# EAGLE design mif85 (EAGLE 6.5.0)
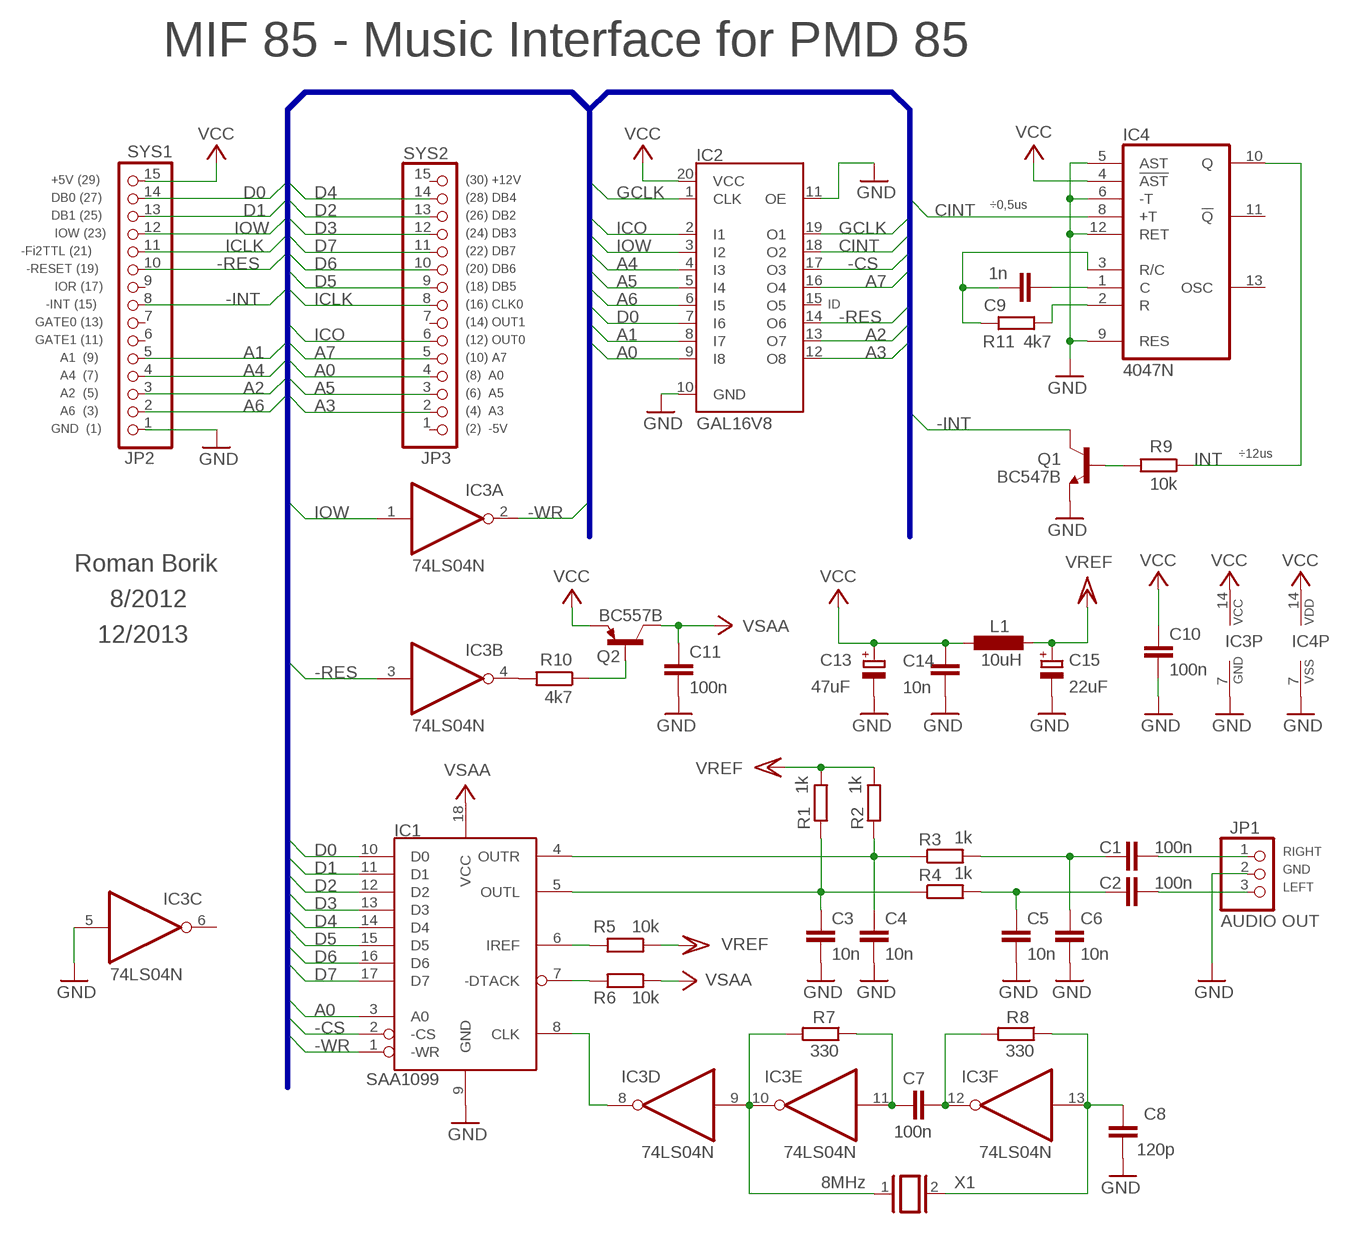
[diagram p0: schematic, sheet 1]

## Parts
C1  100n  C-EU025-025X050  [C025-025X050]
C2  100n  C-EU025-025X050  [C025-025X050]
C3  10n  C-EU025-025X050  [C025-025X050]
C4  10n  C-EU025-025X050  [C025-025X050]
C5  10n  C-EU025-025X050  [C025-025X050]
C6  10n  C-EU025-025X050  [C025-025X050]
C7  100n  C-EU025-025X050  [C025-025X050]
C8  120p  C-EU025-025X050  [C025-025X050]
C9  1n  C-EU025-025X050  [C025-025X050]
C10  100n  C-EU025-025X050  [C025-025X050]
C11  100n  C-EU025-025X050  [C025-025X050]
C13  47uF  CPOL-EUE2,5-6E  [E2,5-6E]
C14  10n  C-EU025-025X050  [C025-025X050]
C15  22uF  CPOL-EUE2,5-6E  [E2,5-6E]
IC1  SAA1099  [DIL18]
IC2  GAL16V8  ATF16V8BP3  [DIL20]
IC3  74LS04N  [DIL14]
IC4  4047N  [DIL14]
JP1  AUDIO OUT  PINHD-1X3  [1X03]
JP2  SYS1  PINHD-1X15  [1X15]
JP3  SYS2  PINHD-1X15  [1X15]
L1  10uH  L-EU0207/7  [0207/7]
Q1  BC547B  [TO92]
Q2  BC557B  BC557  [TO92]
R1  1k  R-EU_0207/7  [0207/7]
R2  1k  R-EU_0207/7  [0207/7]
R3  1k  R-EU_0207/7  [0207/7]
R4  1k  R-EU_0207/7  [0207/7]
R5  10k  R-EU_0207/7  [0207/7]
R6  10k  R-EU_0207/7  [0207/7]
R7  330  R-EU_0207/7  [0207/7]
R8  330  R-EU_0207/7  [0207/7]
R9  10k  R-EU_0207/7  [0207/7]
R10  4k7  R-EU_0207/7  [0207/7]
R11  4k7  R-EU_0207/7  [0207/7]
X1  8MHz  XTAL/S  [QS]

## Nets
-CS: IC1.2(-CS) IC2.17(O3)
-INT: JP2.8 Q1.3(C)
-RES: IC2.14(O6) IC3.3(B:I) JP2.10
-WR: IC1.1(-WR) IC3.2(A:O)
A0: IC1.3(A0) IC2.9(I8) JP3.4
A1: IC2.8(I7) JP2.5
A2: IC2.13(O7) JP2.3
A3: IC2.12(O8) JP3.2
A4: IC2.4(I3) JP2.4
A5: IC2.5(I4) JP3.3
A6: IC2.6(I5) JP2.2
A7: IC2.16(O4) JP3.5
CINT: IC2.18(O2) IC4.8(+T)
D0: IC1.10(D0) IC2.7(I6) JP2.14
D1: IC1.11(D1) JP2.13
D2: IC1.12(D2) JP3.13
D3: IC1.13(D3) JP3.12
D4: IC1.14(D4) JP3.14
D5: IC1.15(D5) JP3.9
D6: IC1.16(D6) JP3.10
D7: IC1.17(D7) JP3.11
GCLK: IC2.1(CLK) IC2.19(O1)
GND: C3.2 C4.2 C5.2 C6.2 C8.2 C10.2 C11.2 C13.- C14.2 C15.- IC1.9(GND) IC2.10(GND) IC2.11(OE) IC3.5(C:I) IC3.7(P:GND) IC4.5(AST) IC4.6(-T) IC4.7(VSS) IC4.9(RES) IC4.12(RET) JP1.2 JP2.1 Q1.1(E)
ICLK: JP2.11 JP3.8
ICO: IC2.2(I1) JP3.6
INT: IC4.10(Q) R9.2
IOW: IC2.3(I2) IC3.1(A:I) JP2.12
N$1: IC3.9(D:I) IC3.10(E:O) R7.2 X1.1
N$2: C7.1 IC3.12(F:O) R8.2
N$3: C7.2 IC3.11(E:I) R7.1
N$4: Q1.2(B) R9.1
N$5: C8.1 IC3.13(F:I) R8.1 X1.2
N$6: IC1.8(CLK) IC3.8(D:O)
N$7: IC4.2(R) R11.2
N$8: IC3.4(B:O) R10.2
N$9: Q2.2(B) R10.1
N$10: IC1.7(-DTACK) R6.2
N$11: IC1.6(IREF) R5.2
N$12: C4.1 IC1.4(OUTR) R2.1 R3.1
N$13: C3.1 IC1.5(OUTL) R1.1 R4.1
N$14: C2.1 C5.1 R4.2
N$15: C1.1 C6.1 R3.2
N$16: C2.2 JP1.3
N$17: C1.2 JP1.1
N$18: C9.2 IC4.1(C)
N$19: C9.1 IC4.3(R/C) R11.1
V+: C11.1 IC1.18(VCC) Q2.3(C) R6.1 ; supply symbol labelled VSAA
VCC: C10.1 C13.+ C14.1 IC2.20(VCC) IC3.14(P:VCC) IC4.4(!AST) IC4.14(VDD) JP2.15 L1.2 Q2.1(E)
VREF: C15.+ L1.1 R1.2 R2.2 R5.1
Unconnected: IC2.15(O5) IC3.6(C:O) IC4.11(!Q) IC4.13(OSC) JP2.6 JP2.7 JP2.9 JP3.1 JP3.7 JP3.15

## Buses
SYS:D[0..7],A[0..7],IOW,-INT,-RES,ICO,ICLK,GCLK,-CS,-WR,CINT

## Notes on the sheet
- MIF 85 - Music Interface for PMD 85
- +5V (29) | (30) +12V
- DB0 (27) | (28) DB4
- ÷0,5us
- DB1 (25) | (26) DB2
- IOW (23) | (24) DB3
- -Fi2TTL (21) | (22) DB7
- -RESET (19) | (20) DB6
- IOR (17) | (18) DB5
- -INT (15) | (16) CLK0 | ID
- GATE0 (13) | (14) OUT1
- GATE1 (11) | (12) OUT0
- A1  (9) | (10) A7
- A4  (7) | (8)  A0
- A2  (5) | (6)  A5
- A6  (3) | (4)  A3
- GND  (1) | (2)  -5V
- ÷12us
- Roman Borik
- 8/2012
- 12/2013
- RIGHT
- GND
- LEFT

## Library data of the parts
C1-C11 C14 = rcl:C-EU: CAPACITOR, European symbol
C13 C15 = rcl:CPOL-EU: POLARIZED CAPACITOR, European symbol
IC1 = rombor:SAA1099
IC2 = atmel:ATF16V8B: High perfomance CMOS (electrically erasable) programmable logic device (PLD) ABLE-Atmel-ABEL - P18V8R, P16V8C, P16V8AS, P17V8 COPL Atmel-WinCUPL - G16V8MS, G16V8MA, G16V8AS, G16V8 LOG/IC - GAL16V8_R, GAL16V8_G7, GAL16V8_C), GAL16V8 Tango-PLD - G16V8R, G16V8C, G16V8AS, G16V8 Source: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; MPN: ATF16V8CZ-15PU; OC_FARNELL: 1551768; OC_NEWARK: 94M6254
IC3 = 74xx-eu:74*04: Hex INVERTER
IC4 = 40xx:4047: LP monostable/astable MULTIVIBRATOR
JP1 = pinhead:PINHD-1X3: PIN HEADER
JP2 JP3 = pinhead:PINHD-1X15: PIN HEADER
L1 = rcl:L-EU: INDUCTOR, European symbol
Q1 = transistor-npn:BC547*: NPN Transistor
Q2 = transistor-pnp:BC557: PNP Transistor
R1-R11 = rcl:R-EU_: RESISTOR, European symbol
X1 = special:XTAL/S: CRYSTAL

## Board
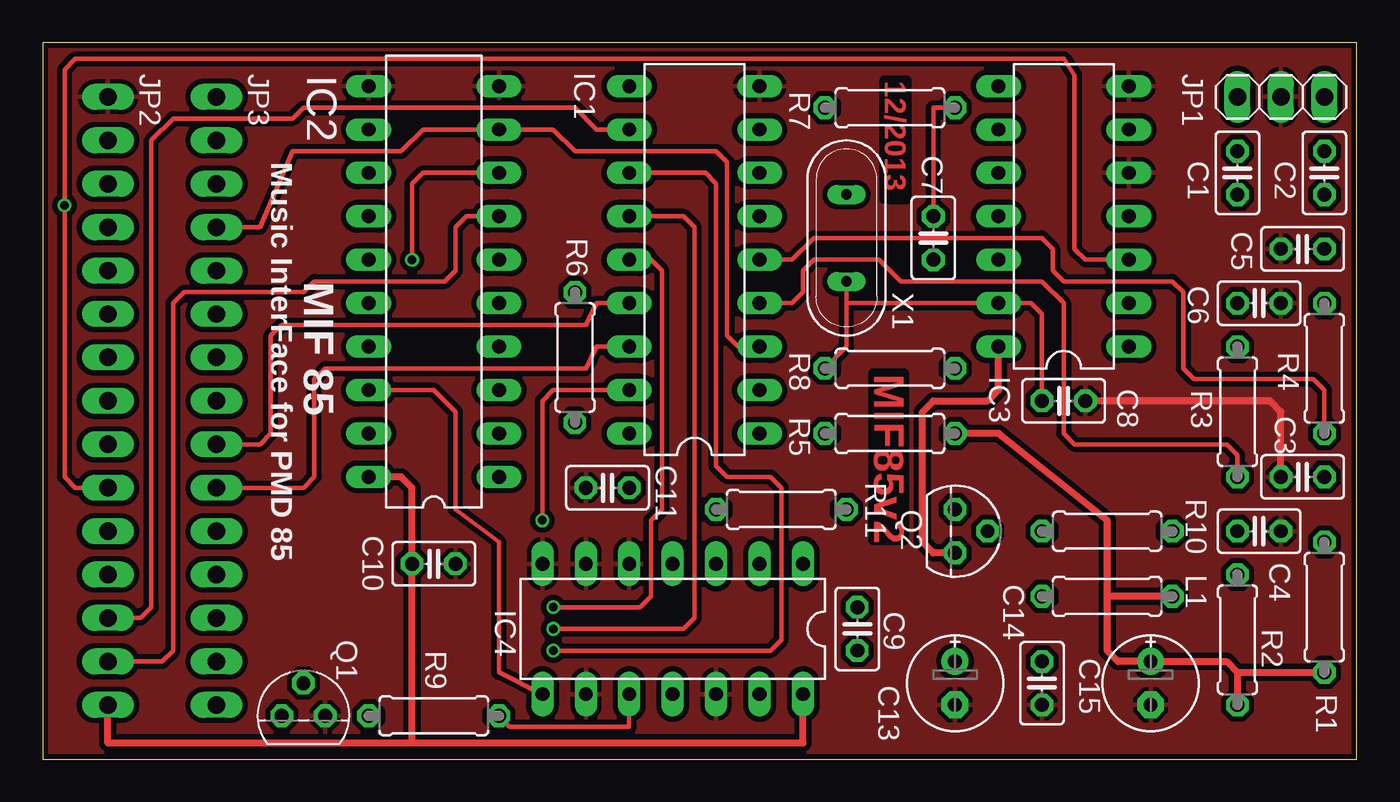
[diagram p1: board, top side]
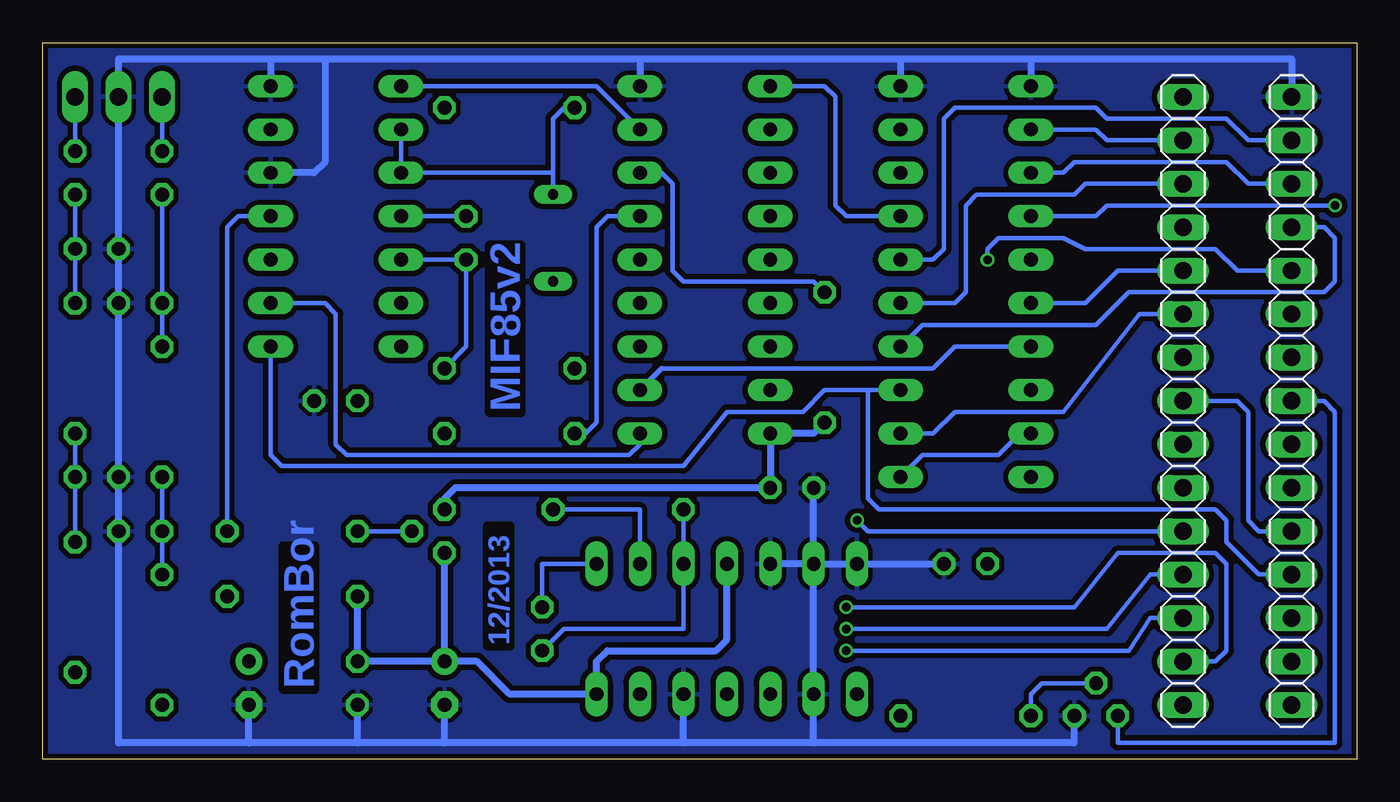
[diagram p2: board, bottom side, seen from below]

Size 76.82 x 41.9 mm. Coordinates in mm from the lower left corner, seen from the top.
Outline: 0,0 76.82,0 76.82,41.9 0,41.9 0,0
Copper layers (1*16): Top 0.035mm / dielectric 1.5mm / Bottom 0.035mm
Design rules "SeeedStudio_2layer_DRU_no_angle_20140221": minimum track width 6mil, minimum drill 12mil, track to track 6mil, track to pad 6mil, pad to pad 6mil, via to via 6mil, smd to smd 0mil, copper to edge 10mil, drill to drill 10mil, minimum pad ring 10mil, minimum via ring 6mil, stop-mask expansion 2mil, vias tented up to drill 100mil, thermal gap 10mil

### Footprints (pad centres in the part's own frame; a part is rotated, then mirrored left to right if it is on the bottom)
C025-025X050 = drill 0.813 octagon: 1 -1.27,0; 2 1.27,0
E2,5-6E = drill 0.813 pad 1.575: + -1.27,0 | drill 0.813 pad 1.575 octagon: - 1.27,0
DIL18 = drill 0.813 long: 1 -10.16,-3.81; 2 -7.62,-3.81; 3 -5.08,-3.81; 4 -2.54,-3.81; 5 0,-3.81; 6 2.54,-3.81; 7 5.08,-3.81; 8 7.62,-3.81; 9 10.16,-3.81; 10 10.16,3.81; 11 7.62,3.81; 12 5.08,3.81; 13 2.54,3.81; 14 0,3.81; 15 -2.54,3.81; 16 -5.08,3.81; 17 -7.62,3.81; 18 -10.16,3.81
DIL20 = drill 0.813 long: 1 -11.43,-3.81; 2 -8.89,-3.81; 3 -6.35,-3.81; 4 -3.81,-3.81; 5 -1.27,-3.81; 6 1.27,-3.81; 7 3.81,-3.81; 8 6.35,-3.81; 9 8.89,-3.81; 10 11.43,-3.81; 11 11.43,3.81; 12 8.89,3.81; 13 6.35,3.81; 14 3.81,3.81; 15 1.27,3.81; 16 -1.27,3.81; 17 -3.81,3.81; 18 -6.35,3.81; 19 -8.89,3.81; 20 -11.43,3.81
DIL14 = drill 0.813 long: 1 -7.62,-3.81; 2 -5.08,-3.81; 3 -2.54,-3.81; 4 0,-3.81; 5 2.54,-3.81; 6 5.08,-3.81; 7 7.62,-3.81; 8 7.62,3.81; 9 5.08,3.81; 10 2.54,3.81; 11 0,3.81; 12 -2.54,3.81; 13 -5.08,3.81; 14 -7.62,3.81
1X03 = drill 1.016 long: 1 -2.54,0; 2 0,0; 3 2.54,0
1X15 = drill 1.016 long: 1 -17.78,0; 2 -15.24,0; 3 -12.7,0; 4 -10.16,0; 5 -7.62,0; 6 -5.08,0; 7 -2.54,0; 8 0,0; 9 2.54,0; 10 5.08,0; 11 7.62,0; 12 10.16,0; 13 12.7,0; 14 15.24,0; 15 17.78,0
0207/7 = drill 0.813 octagon: 1 -3.81,0; 2 3.81,0
TO92 = drill 0.813 octagon: 1 1.27,0; 2 0,1.905; 3 -1.27,0
QS = drill 0.61 long: 1 -2.54,0; 2 2.54,0

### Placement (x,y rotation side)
C1  69.85,34.29 90 top
C2  74.93,34.29 90 top
C3  73.66,16.51 180 top
C4  71.12,13.34 0 top
C5  73.66,29.84 180 top
C6  71.12,26.67 0 top
C7  52.07,30.48 90 top
C8  59.69,20.95 0 top
C9  47.62,7.62 90 top
C10  22.86,11.43 0 top
C11  33.02,15.88 180 top
C13  53.34,4.45 270 top
C14  58.42,4.45 270 top
C15  64.77,4.45 270 top
IC1  38.1,29.21 90 top
IC2  22.86,27.94 90 top
IC3  59.69,31.75 90 top
IC4  36.83,7.62 180 top
JP1  72.39,38.73 0 top
JP2  3.81,20.95 270 bottom
JP3  10.16,20.95 270 bottom
L1  62.23,9.53 180 top
Q1  15.24,2.54 0 top
Q2  53.34,13.34 270 top
R1  74.93,8.89 270 top
R2  69.85,6.99 270 top
R3  69.85,20.32 90 top
R4  74.93,22.86 90 top
R5  49.53,19.05 180 top
R6  31.11,23.5 90 top
R7  49.53,38.1 180 top
R8  49.53,22.86 0 top
R9  22.86,2.54 0 top
R10  62.23,13.34 0 top
R11  43.18,14.61 0 top
X1  46.99,30.48 270 top

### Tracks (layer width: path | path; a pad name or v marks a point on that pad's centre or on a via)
-CS
  Bottom 0.254: IC2.17 23.5,24.13 24.77,22.86 40.64,22.86
  Bottom 0.305: 40.64,22.86 IC1.2
-INT
  Bottom 0.254: JP2.8 1.91,20.95 1.27,20.32 1.27,0.95 13.97,0.95 Q1.3
-RES  (via drill 0.5)
  Top 0.254: IC3.3 60.96,29.21 60.33,29.84 60.33,40.01 59.69,40.96 1.91,40.96 1.27,40.32 v1.27,32.38 1.27,16.51 1.91,15.88 JP2.10
  Bottom 0.254: IC2.14 15.24,31.75 14.61,32.38 v1.27,32.38
-WR
  Bottom 0.254: IC1.1 41.91,18.41 42.55,17.78 59.05,17.78 59.69,18.41 59.69,26.04 60.33,26.67 IC3.2
A0
  Top 0.254: JP3.4 12.7,31.11 14.61,35.56 20.95,35.56 22.23,36.83 IC2.9 29.84,36.83 31.11,35.56 39.37,35.56 40.01,34.92 40.01,24.77 40.64,24.13 IC1.3
A1  (via drill 0.5)
  Top 0.254: v21.59,29.21 21.59,33.66 22.23,34.29 IC2.8
  Bottom 0.254: v21.59,29.21 21.59,29.84 20.95,30.48 17.14,30.48 15.88,29.84 8.26,29.84 6.99,28.57 JP2.5
A2
  Bottom 0.254: JP2.3 6.35,33.66 7.62,34.92 16.51,34.92 17.14,34.29 IC2.13
A3
  Bottom 0.254: JP3.2 14.61,36.2 15.24,36.83 IC2.12
A4
  Bottom 0.254: JP2.4 1.91,31.11 1.27,30.48 1.27,27.94 1.91,27.3 13.34,27.3 15.24,25.4 25.4,25.4 IC2.4
A5
  Bottom 0.254: IC2.5 23.5,26.67 22.86,27.3 22.86,32.38 22.23,33.02 16.51,33.02 15.88,33.66 JP3.3
A6
  Bottom 0.254: JP2.2 6.35,36.2 7.62,37.47 14.61,37.47 15.24,38.1 23.5,38.1 24.13,37.47 24.13,29.84 24.77,29.21 IC2.6
A7
  Bottom 0.254: JP3.5 13.97,28.57 15.88,26.67 IC2.16
CINT
  Top 0.254: IC4.8 26.67,5.08 26.67,12.7 24.13,14.61 24.13,20.32 22.86,21.59 IC2.18
D0
  Top 0.254: IC2.7 24.77,31.75 24.13,31.11 24.13,28.57 23.5,27.94 15.88,27.94 15.24,27.3 8.26,27.3 7.62,26.67 7.62,6.35 6.99,5.71 JP2.14
  Bottom 0.254: IC1.10 31.11,39.37 30.48,38.73 30.48,32.38 29.84,31.75 IC2.7
D1
  Top 0.254: IC1.11 32.38,36.83 31.11,38.1 15.24,38.1 14.61,37.47 7.62,37.47 6.35,36.2 6.35,8.89 5.71,8.26 JP2.13
D2  (via drill 0.5)
  Top 0.254: IC1.12 38.73,34.29 39.37,33.66 39.37,17.14 40.01,16.51 42.55,16.51 43.18,15.88 43.18,6.99 42.55,6.35 v29.84,6.35
  Bottom 0.254: v29.84,6.35 13.34,6.35 12.06,8.26 JP3.13
D3  (via drill 0.5)
  Top 0.254: IC1.13 37.47,31.75 38.1,31.11 38.1,8.26 37.47,7.62 v29.84,7.62
  Bottom 0.254: v29.84,7.62 14.61,7.62 12.06,10.79 JP3.12
D4  (via drill 0.5)
  Top 0.254: 35.56,29.21 36.2,28.57 36.2,14.61 35.56,13.97 35.56,9.53 34.92,8.89 v29.84,8.89
  Top 0.305: 35.56,29.21 IC1.14
  Bottom 0.254: v29.84,8.89 16.51,8.89 13.97,12.06 8.26,12.06 7.62,11.43 7.62,6.35 8.26,5.71 JP3.14
D5
  Top 0.254: IC1.15 32.38,26.67 31.75,25.4 13.97,25.4 13.34,24.77 13.34,19.05 12.7,18.41 JP3.9
D6
  Top 0.254: IC1.16 32.38,24.13 31.75,22.86 16.51,22.86 15.88,22.23 15.88,16.51 15.24,15.88 JP3.10
D7  (via drill 0.5)
  Top 0.254: IC1.17 29.84,21.59 29.21,20.95 v29.21,13.97
  Bottom 0.254: v29.21,13.97 28.57,13.34 JP3.11
GCLK
  Bottom 0.254: IC2.1 25.4,17.78 20.95,17.78 19.68,19.05 IC2.19
GND
  Top 0.406: C8.2 71.75,20.95 72.39,20.32 C3.2
  Bottom 0.406: 64.77,0.95 72.39,0.95 C4.2 C3.2 C6.2 C5.2 JP1.2 72.39,40.96 63.5,40.96 | 63.5,40.96 IC3.7 | 63.5,40.96 60.33,40.96 | 60.33,40.96 60.33,34.92 60.96,34.29 IC3.5 | 60.33,40.96 41.91,40.96 | 41.91,40.96 IC1.9 | 41.91,40.96 26.67,40.96 | 26.67,40.96 IC2.10 | 26.67,40.96 19.05,40.96 | 19.05,40.96 IC2.11 | 19.05,40.96 3.81,40.96 JP2.1 | 64.77,0.95 C15.- | 58.42,0.95 64.77,0.95 | 58.42,0.95 C14.2 | 53.34,0.95 58.42,0.95 | 53.34,0.95 C13.- | 39.37,0.95 53.34,0.95 | 39.37,0.95 IC4.12 | 31.75,0.95 39.37,0.95 | IC4.6 IC4.5 | IC4.6 IC4.7 C10.2 | IC4.6 C11.2 | IC4.6 IC4.9 31.75,0.95 | 31.75,0.95 16.51,0.95 Q1.1
  pour Top (isolate 0.305): 0,41.91 76.83,41.91 76.83,0 0,0
  pour Bottom (isolate 0.305): 0,41.91 76.83,41.91 76.83,0 0,0
ICLK
  Bottom 0.254: JP2.11 5.71,13.34 6.35,13.97 6.35,20.32 6.99,20.95 JP3.8
ICO
  Bottom 0.254: JP3.6 12.7,26.04 17.14,20.32 23.5,20.32 24.77,19.05 IC2.2
INT
  Top 0.254: R9.2 27.3,1.91 34.29,1.91 IC4.10
IOW
  Bottom 0.254: IC3.1 63.5,17.78 62.87,17.14 39.37,17.14 36.83,20.32 32.38,20.32 31.11,21.59 28.57,21.59 | 28.57,21.59 IC2.3 | JP2.12 5.71,10.79 7.62,12.7 7.62,13.97 8.26,14.61 27.94,14.61 28.57,15.24 28.57,21.59
N$1
  Bottom 0.254: IC3.9 IC3.10 46.99,34.29 | R7.2 46.35,38.1 46.99,37.47 46.99,34.29 | X1.1 46.99,34.29
N$2
  Bottom 0.254: IC3.12 C7.1 52.07,24.13 R8.2
N$3
  Top 0.254: C7.2 52.07,38.1 R7.1
  Bottom 0.254: C7.2 IC3.11
N$4
  Bottom 0.254: R9.1 19.05,3.81 18.41,4.45 Q1.2
N$5
  Top 0.254: R8.1 46.99,24.13 46.99,26.67 | 46.99,26.67 X1.2 | 46.99,26.67 IC3.13 57.78,26.67 58.42,26.04 C8.1
N$6
  Bottom 0.254: IC3.8 44.45,39.37 IC1.8
N$7
  Bottom 0.254: IC4.2 41.91,14.61 R11.2
N$8
  Bottom 0.254: R10.2 66.04,31.11 65.41,31.75 IC3.4
N$9
  Bottom 0.254: Q2.2 R10.1
N$10
  Bottom 0.254: R6.2 31.75,27.94 39.37,27.94 40.01,28.57 40.01,33.66 40.64,34.29 IC1.7
N$11
  Bottom 0.254: R5.2 45.09,19.05 44.45,19.68 44.45,31.11 43.81,31.75 IC1.6
N$12
  Top 0.254: R3.1 69.85,17.78 69.22,18.41 60.33,18.41 59.69,19.05 59.69,26.67 58.42,27.94 50.16,27.94 48.9,29.21 45.09,29.21 44.45,28.57 44.45,27.3 43.81,26.67 IC1.4
  Bottom 0.254: R2.1 C4.1 R3.1
N$13
  Top 0.254: IC1.5 43.81,29.21 45.09,30.48 58.42,30.48 59.05,29.84 59.05,28.57 59.69,27.94 66.04,27.94 66.67,27.3 66.67,22.86 67.31,22.23 74.3,22.23 74.93,21.59 R4.1
  Bottom 0.254: R4.1 C3.1 R1.1
N$14
  Bottom 0.254: C2.1 C5.1 R4.2
N$15
  Bottom 0.254: C1.1 C6.1 R3.2
N$16
  Bottom 0.254: C2.2 JP1.3
N$17
  Bottom 0.254: C1.2 JP1.1
N$18
  Bottom 0.254: C9.2 47.62,11.43 IC4.1
N$19
  Bottom 0.254: R11.1 IC4.3 39.37,7.62 46.35,7.62 C9.1
V+
  Bottom 0.406: Q2.3 53.34,15.24 52.7,15.88 C11.1 IC1.18 31.75,19.05 R6.1
VCC
  Top 0.406: JP2.15 3.81,0.95 21.59,0.95 | 21.59,0.95 44.45,0.95 IC4.14 | 21.59,0.95 C10.1 21.59,15.88 20.95,16.51 IC2.20 | Q2.1 52.07,12.06 51.44,12.7 51.44,20.32 52.07,20.95 55.24,20.95 55.88,21.59 IC3.14
  Bottom 0.406: IC4.4 36.83,6.99 37.47,6.35 43.81,6.35 44.45,5.71 IC4.14 49.53,3.81 51.44,5.71 C13.+ | C13.+ C14.1 L1.2 | C13.+ Q2.1
VREF
  Top 0.406: 69.85,5.08 R1.2 | 69.85,5.08 69.22,5.71 C15.+ 62.87,5.71 62.23,6.35 62.23,9.53 | 69.85,5.08 R2.2 | 62.23,9.53 62.23,13.97 55.88,19.05 R5.1 | L1.1 62.23,9.53

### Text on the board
Top: 12/2013 | MIF85v2
Bottom: MIF85v2 | 12/2013 | RomBor
tPlace: MIF 85
tNames: Music InterFace for PMD 85
Document: JP2 a JP3 sa osadzuju na stranu spojov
